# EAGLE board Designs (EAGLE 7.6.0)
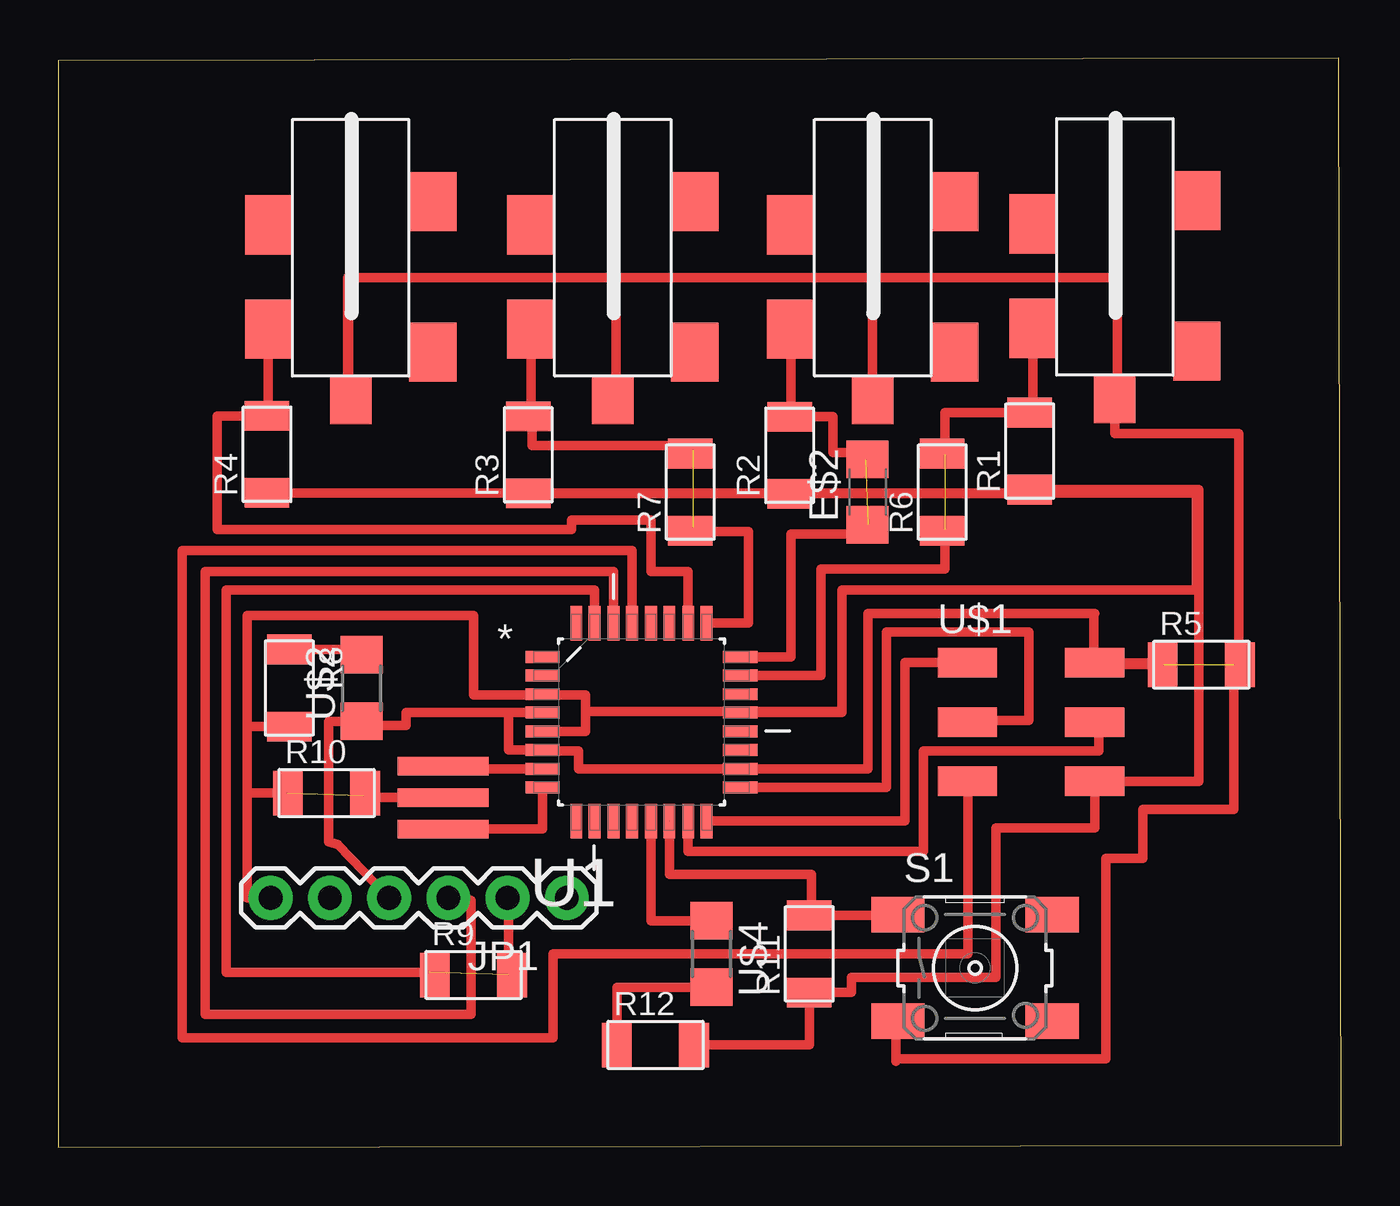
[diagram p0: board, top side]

Size 55 x 46.7 mm. Coordinates in mm from the lower left corner, seen from the top.
Outline: 0,0 55,0.1 54.9,46.7 0,46.6 0,0
Copper layers (1*16): Top 0.035mm / dielectric 1.5mm / Bottom 0.035mm
Design rules "default": minimum track width 10mil, minimum drill 24mil, track to track 8mil, track to pad 8mil, pad to pad 8mil, via to via 8mil, smd to smd 8mil, copper to edge 40mil, drill to drill 8mil, minimum pad ring 10mil, minimum via ring 8mil, stop-mask expansion 4mil, vias tented up to drill 0mil, thermal gap 10mil

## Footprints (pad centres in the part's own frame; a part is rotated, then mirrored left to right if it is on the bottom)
C1206 = smd 1.6 x 1.8: 1 -1.4,0; 2 1.4,0
JACK_.65MM = smd 2.032 x 2.54: CONTACT 3.578,4.026; SHIELD -3.45,-1.448; SHIELD1 3.578,-0.447; SHUNT -3.45,5.005 | smd 1.778 x 2.032: PIN 0.064,7.071
FTDI_BASIC = drill 1.016 pad 1.88: CTS 10.16,0; DTR 0,0; GND 12.7,0; RXI 2.54,0; TXO 5.08,0; VCC 7.62,0
R1206FAB = smd 1.27 x 1.905: 1 -1.651,0; 2 1.651,0
6MM_SWITCH = smd 2.286 x 1.524: 1 -3.302,2.286; 2 3.302,2.286; 3 -3.302,-2.286; 4 3.302,-2.286
QFP80P900X900X120-32N = smd 1.473 x 0.508: 1 -4.242,2.794; 2 -4.242,2.007; 3 -4.242,1.194; 4 -4.242,0.406; 5 -4.242,-0.406; 6 -4.242,-1.194; 7 -4.242,-2.007; 8 -4.242,-2.794; 17 4.242,-2.794; 18 4.242,-2.007; 19 4.242,-1.194; 20 4.242,-0.406; 21 4.242,0.406; 22 4.242,1.194; 23 4.242,2.007; 24 4.242,2.794 | smd 0.508 x 1.473: 9 -2.794,-4.242; 10 -2.007,-4.242; 11 -1.194,-4.242; 12 -0.406,-4.242; 13 0.406,-4.242; 14 1.194,-4.242; 15 2.007,-4.242; 16 2.794,-4.242; 25 2.794,4.242; 26 2.007,4.242; 27 1.194,4.242; 28 0.406,4.242; 29 -0.406,4.242; 30 -1.194,4.242; 31 -2.007,4.242; 32 -2.794,4.242
2X03SMD = smd 2.54 x 1.27: 1 -2.54,2.54; 2 2.92,2.54; 3 -2.54,0; 4 2.92,0; 5 -2.54,-2.54; 6 2.92,-2.54
1206 = smd 1.6 x 1.803: 1 -1.422,0; 2 1.422,0
EFOBM = smd 0.8 x 3.9: 1 -1.35,0; 2 0,0; 3 1.35,0

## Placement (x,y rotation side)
E$2  [C1206]  34.7,28.1 90 top
J1  JACK.65MM  [JACK_.65MM]  45.36,39.15 180 top
J2  JACK.65MM  [JACK_.65MM]  34.98,39.11 180 top
J3  JACK.65MM  [JACK_.65MM]  23.84,39.11 180 top
J4  JACK.65MM  [JACK_.65MM]  12.6,39.11 180 top
JP1  FTDI_BASICPTH  [FTDI_BASIC]  21.8,10.7 180 top
R1  [R1206FAB]  41.65,29.86 90 top
R2  [R1206FAB]  31.35,29.68 90 top
R3  [R1206FAB]  20.15,29.7 90 top
R4  [R1206FAB]  8.95,29.72 90 top
R5  [R1206FAB]  49,20.7 0 top
R6  [R1206FAB]  37.9,28.1 90 top
R7  [R1206FAB]  27.1,28.1 90 top
R8  [R1206FAB]  9.9,19.7 270 top
R9  [R1206FAB]  17.8,7.4 0 top
R10  [R1206FAB]  11.5,15.2 0 top
R11  [R1206FAB]  32.2,8.3 90 top
R12  [R1206FAB]  25.6,4.4 0 top
S1  [6MM_SWITCH]  39.3,7.7 0 top
U1  ATMEGA328P-AU  [QFP80P900X900X120-32N]  25,18.24 0 top
U$1  AVRISPSMD  [2X03SMD]  41.51,18.24 0 top
U$2  [1206]  13,19.7 90 top
U$3  RESONATOR  [EFOBM]  16.5,15 270 top
U$4  [1206]  28,8.3 270 top

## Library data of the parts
E$2 = resistor
J1-J4 R1-R12 S1 U$1 U$3 = fab
JP1 = SparkFun
U1 = Atmel-ATMEGA328P-AU; DESCRIPTION: 8-bit Microcontroller with In-System Programmable Flash; MPN: ATMEGA328P-AU; OC_FARNELL: 1715486; OC_NEWARK: 14R4631; PACKAGE: TQFP-32; SUPPLIER: Atmel
U$2 U$4 = FabLab

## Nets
N$1: R5.1 U$1.2
N$3: U1.15 U$1.4
N$4: U1.16 U$1.1
N$5: U1.29 U$1.5
N$6: U1.17 U$1.3
N$7: JP1.GND R1.1 R2.1 R3.1 R4.1 R8.2 R11.1 R12.2 U1.3 U1.5 U1.21 U$1.6 U$3.2
N$8: J1.CONTACT R1.2 U1.23
N$9: J2.CONTACT R2.2 U1.24
N$10: J3.CONTACT R3.2 U1.25
N$11: J4.CONTACT R4.2 U1.26
N$13: J1.PIN J2.PIN J3.PIN J4.PIN JP1.VCC R5.2 S1.3 U1.4 U1.6 U1.18 U$2.1
N$14: JP1.TXO U1.30
N$15: JP1.RXI U1.31
N$16: R8.1 U$2.2
N$17: U1.7 U$3.1
N$18: U1.8 U$3.3
N$19: R11.2 S1.1 U1.14
N$20: R12.1 U$4.2
N$21: U1.13 U$4.1

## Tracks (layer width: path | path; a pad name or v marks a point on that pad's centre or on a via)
N$1
  Top 0.406: U$1.2 47.35,20.78 R5.1
N$3
  Top 0.406: U$1.4 44.6,18.24 44.6,17 37.1,17 37.1,12.7 27,12.7 U1.15
N$4
  Top 0.406: U1.16 36.3,14 36.3,20.8 38.97,20.8 U$1.1
N$5
  Top 0.406: U1.29 24.6,25.6 5.3,25.6 5.3,4.7 21.2,4.7 21.2,8.3 39,8.3 39,15.7 U$1.5
N$6
  Top 0.406: U1.17 35.5,15.45 35.5,22.1 41.6,22.1 41.6,18.3 38.97,18.3 U$1.3
N$7  (1 unrouted)
  Top 0.406: 48.9,23.9 48.9,15.7 U$1.6 44.43,13.7 40.2,13.7 40.2,7.3 34,7.3 34,6.65 R11.1 32.2,4.4 R12.2 | 48.9,23.9 48.9,28.2 R1.1 41.85,28.03 R2.1 31.35,28.05 R3.1 20.15,28.07 R4.1 48.8,28.07 48.8,23.9 | U1.21 33.6,18.65 33.6,18.7 | 48.8,23.9 48.9,23.9 | JP1.GND 8.1,10.7 8.1,15.2 | 8.1,15.2 8.1,18.05 | 20.76,19.4 17.8,19.4 17.8,22.8 8.1,22.8 8.1,18.05 | R8.2 8.1,18.05 | 8.1,15.2 9.8,15.2 | U$3.2 13.1,15 13.1,15.1 | U1.5 22.6,17.83 22.6,18.7 | 22.6,18.7 22.6,19.4 20.76,19.4 | 20.76,19.4 U1.3 | 48.8,23.9 33.6,23.9 33.6,18.7 | 33.6,18.7 22.6,18.7
N$8  (1 unrouted)
  Top 0.406: J1.CONTACT 41.78,31.61 R1.2 38,31.51 38,29.7 | U1.23 32.7,20.25 32.7,24.8 38,24.8 38,26.5
N$9  (1 unrouted)
  Top 0.406: J2.CONTACT 31.4,31.33 R2.2 33.2,31.33 33.2,29.8 34.6,29.8 34.6,29.5 | U1.24 31.4,21.03 31.4,26.3 34.7,26.3 34.7,26.7
N$10  (1 unrouted)
  Top 0.406: J3.CONTACT 20.26,31.35 R3.2 20.3,31.35 20.3,30.1 27.2,30.1 27.2,29.9 | U1.25 29.6,22.48 29.6,26.4 27.2,26.4 27.2,26.6
N$11
  Top 0.406: J4.CONTACT 9,35.08 9,31.37 | 9,31.37 9,31.2 | U1.26 27,24.7 25.4,24.7 25.4,26.9 22,26.9 22,26.5 6.8,26.5 6.8,31.37 R4.2 9,31.37
N$13  (1 unrouted)
  Top 0.406: U1.4 19.3,18.65 | 19.3,18.65 14.9,18.65 14.9,18.1 13,18.1 U$2.1 11.6,18.28 11.6,13.1 11.98,13 JP1.VCC | 44.4,22.9 34.7,22.9 34.7,16.23 U1.18 22.3,16.23 22.3,17 20.76,17 U1.6 19.3,17.05 19.3,18.65 | 45.4,31.88 J1.PIN 45.3,30.6 50.6,30.6 50.6,20.7 R5.2 50.4,20.7 50.4,14.5 46.5,14.5 46.5,12.4 44.9,12.4 44.9,3.8 35.9,3.8 | 34.9,37.3 45.4,37.3 45.4,31.88 | 34.9,37.3 23.9,37.3 | 23.9,37.3 12.44,37.3 | 12.44,37.3 12.44,32.04 J4.PIN 12.4,32.04 12.4,37.3 12.44,37.3 | J3.PIN 23.9,32.04 23.9,37.3 | J2.PIN 34.9,32.04 34.9,37.3 | 45.4,31.88 45.43,31.88 | 44.43,22.9 44.4,22.9 | 44.4,22.9 44.4,20.7 47.4,20.7 | S1.3 35.9,5.41 35.9,3.8 | 35.9,3.8 35.9,3.7
N$14
  Top 0.406: JP1.TXO 17.7,10.6 17.7,5.7 6.3,5.7 6.3,24.7 23.81,24.7 U1.30
N$15  (1 unrouted)
  Top 0.406: U1.31 23,23.9 7.2,23.9 7.2,7.5 15.9,7.5 | JP1.RXI 19.3,10.7 19.3,7.4
N$16
  Top 0.406: 13.6,21.35 U$2.2 13,21.35 R8.1
N$17
  Top 0.406: U1.7 17.3,16.23 U$3.1
N$18
  Top 0.406: U$3.3 20.76,13.65 U1.8
N$19  (1 unrouted)
  Top 0.406: S1.1 36,9.95 R11.2 32.3,9.95 32.3,11.7 26.2,11.7 U1.14
N$20
  Top 0.406: U$4.2 23.95,6.88 R12.1
N$21
  Top 0.406: U$4.1 25.41,9.72 U1.13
